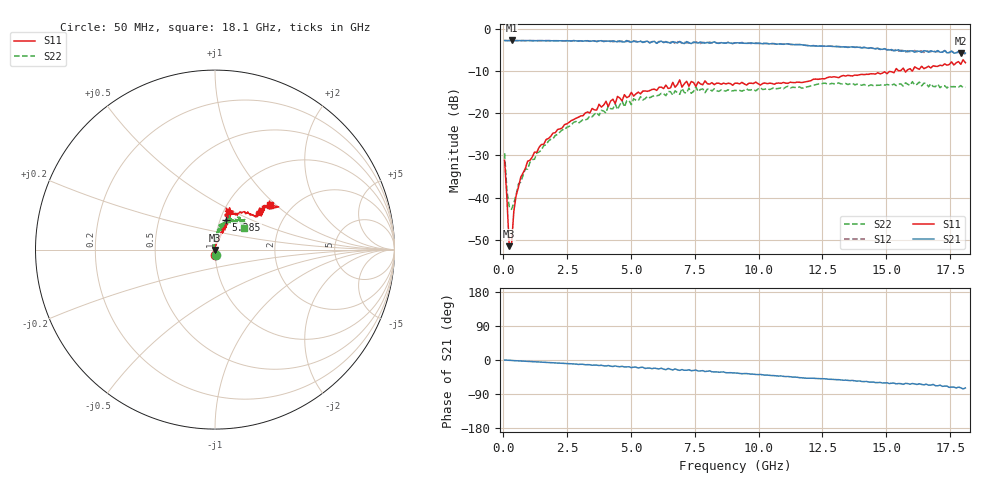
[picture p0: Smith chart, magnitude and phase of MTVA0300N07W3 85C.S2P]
! Network Analyzer HP8720D.06.14 Serial No. US36140669
!  7 Jul 2005  12:02:20
! Frequency  S11  S21  S12  S22
# HZ  S  DB R 50
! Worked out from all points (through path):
!   201 points, 50 MHz to 18.1 GHz, reference 50 ohm
!   highest |S21| = -2.82 dB at 320.8 MHz (marker M1); lowest = -5.9 dB at 17.92 GHz (marker M2)
!   group delay of S21, straight-line fit = 11.3 ps
!   lowest |S11| = -51.5 dB at 230.5 MHz (marker M3), VSWR 1.01, Z = 49.9 - j0.256 ohm
!   |S11| at or under -10 dB: start of sweep to 15.34 GHz; 15.48208 GHz to 15.48747 GHz (5.385 MHz wide, 0.0348 % of centre); 15.72552 GHz to 15.79991 GHz (74.39 MHz wide, 0.472 % of centre)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
!   |S22| runs from -42.8 to -12.6 dB; largest |S21 - S12| = 0.04
!   S11 on the Smith chart (normalised r, x): 50 MHz: 1.00, -0.06; 5.285 GHz: 1.07, +0.36; 18.1 GHz: 1.56, +0.92
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5e7  -31.17 -84.8  -2.82 0.0  -2.81 0.1  -29.51 -78.0
1.4025e8  -40.19 -91.3  -2.87 -0.5  -2.85 -0.5  -38.33 -120.5
2.305e8  -51.50 -105.2  -2.84 -0.8  -2.83 -0.8  -42.17 -152.3
3.2075e8  -51.14 108.9  -2.82 -1.0  -2.84 -1.1  -42.79 167.4
4.11e8  -43.25 92.6  -2.85 -1.6  -2.84 -1.6  -41.26 145.3
5.0125e8  -39.54 91.0  -2.85 -1.9  -2.84 -1.9  -39.36 124.6
5.915e8  -37.55 87.3  -2.85 -2.1  -2.86 -2.2  -36.81 119.8
9.525e8  -31.38 79.5  -2.85 -3.6  -2.84 -3.5  -33.26 103.2
1.76475e9  -26.02 74.7  -2.85 -6.7  -2.86 -6.8  -26.65 87.3
3.1185e9  -20.64 69.1  -2.96 -11.3  -2.98 -11.8  -21.54 84.0
5.2845e9  -15.06 69.5  -3.14 -21.4  -3.20 -20.7  -17.09 69.9
6.09675e9  -13.91 67.2  -3.14 -23.6  -3.05 -23.3  -15.77 69.5
6.7285e9  -13.90 74.0  -3.23 -23.5  -3.51 -24.6  -14.73 63.5
6.909e9  -12.15 70.8  -3.04 -27.4  -3.16 -25.4  -15.57 63.7
6.99925e9  -13.85 70.6  -3.35 -25.3  -3.51 -27.6  -14.15 64.3
7.17975e9  -12.46 74.9  -3.08 -27.0  -3.38 -25.6  -15.26 60.3
7.54075e9  -13.70 67.6  -3.32 -26.4  -3.16 -29.5  -13.77 67.3
9.075e9  -12.93 69.7  -3.39 -34.2  -3.36 -34.4  -14.63 57.8
1.21435e10  -11.99 56.1  -4.07 -48.2  -4.02 -48.3  -13.45 55.5
1.512175e10  -10.14 37.9  -5.06 -62.2  -4.85 -61.6  -13.37 49.3
1.79195e10  -8.46 36.8  -5.85 -73.3  -5.65 -74.3  -13.50 42.5
1.81e10  -8.07 38.9  -5.82 -73.7  -6.11 -74.7  -13.90 36.6
